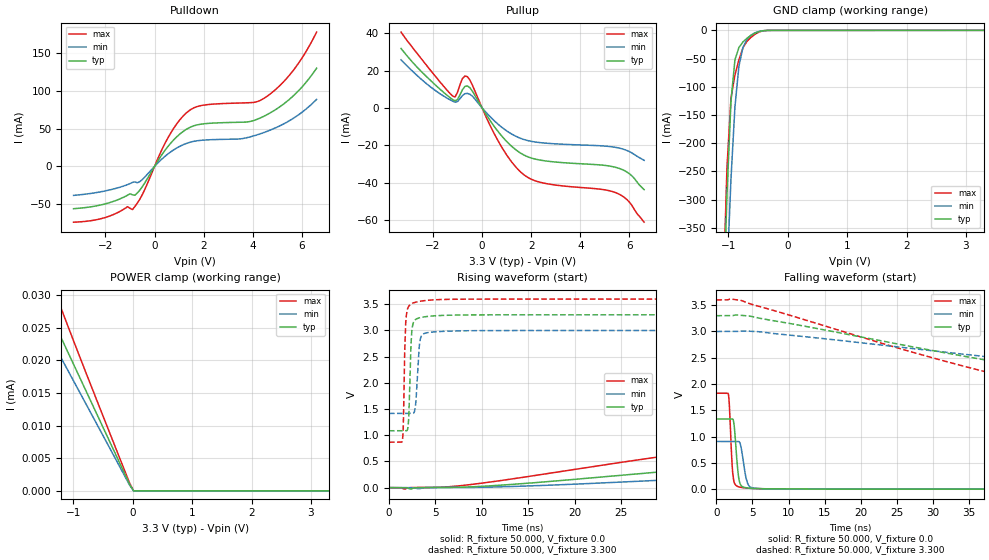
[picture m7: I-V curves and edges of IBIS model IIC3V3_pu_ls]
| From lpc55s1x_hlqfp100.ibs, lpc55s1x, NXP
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|   Model IIC3V3_pu_ls
[Model] IIC3V3_pu_ls
Model_type I/O
Polarity   Non-Inverting
Enable   Active-Low
Vinl =  0.990V
Vinh =  2.310V
Vmeas =  1.650V
Cref =  0.0F
Rref =  100.000
Vref =  0.0V
C_comp   2.367pF   2.322pF   2.392pF
C_comp_pullup   0.515pF   0.425pF   0.587pF
C_comp_pulldown   1.564pF   1.480pF   1.635pF
[Model Spec]
Vinh   2.310V   2.100V   2.520V
Vinl   0.990V   0.900V   1.080V
Vmeas   1.650V   1.500V   1.800V
Vref   0.0V   0.0V   0.0V
Cref   0.0F   0.0F   0.0F
Rref   100.000   100.000   100.000
[Temperature Range]   25.000   0.125k   -40.000
[Voltage Range]   3.300V   3.000V   3.600V
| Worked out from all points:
|   slope of the pulldown table from 0 to 0.495 V, typ, clamps not added: 20.4 ohm
|   slope of the pullup table from 0 to 0.495 V, typ, clamps not added: 49.8 ohm
|   GND clamp passes 1 mA (typ) near -0.43 V on its own axis
|   rising waveform, R_fixture 50.000, V_fixture 0.0: 20-80 % time 64.7ns typ, 78.1ns min, 51.2ns max; typ from 0.001 V to 1.33 V
|   rising waveform, R_fixture 50.000, V_fixture 3.300: 20-80 % time 237ps typ, 323ps min, 201ps max; typ from 1.09 V to 3.3 V
|   falling waveform, R_fixture 50.000, V_fixture 0.0: 20-80 % time 483ps typ, 657ps min, 379ps max; typ from 1.34 V to 0.001 V
|   falling waveform, R_fixture 50.000, V_fixture 3.300: 20-80 % time 50.7ns typ, 68.5ns min, 38.4ns max; typ from 3.3 V to 1.09 V
[Pulldown]
|Voltage   I(typ)   I(min)   I(max)
-3.3V     -56mA      -38.4mA    -73.87mA
-2.1V     -50.37mA   -33.07mA   -68.52mA
-1.1V     -38.15mA   -24.11mA   -53.37mA
-900mV    -37.61mA   -21.16mA   -57.18mA
-500mV    -26.92mA   -17.4mA    -37.43mA
500mV     24.51mA    15.34mA    35.14mA
1.2V      47.07mA    29.16mA    67.89mA
1.9V      55.94mA    34.55mA    80.54mA
3.8V      58.93mA    38.31mA    84.23mA
4.5V      67.15mA    45.39mA    91.04mA
5.6V      91.85mA    62.59mA    125mA
6.6V      130mA      88.72mA    177.8mA
[Pullup]
|Voltage   I(typ)   I(min)   I(max)
-3.3V     31.77mA    25.72mA    40.57mA
-2.2V     15.94mA    12.27mA    21.75mA
-1.2V     4.452mA    3.6mA      6.337mA
-1.1V     3.726mA    3.058mA    5.816mA
-800mV    9.696mA    6.594mA    15.7mA
-600mV    11.73mA    7.748mA    16.71mA
700mV     -13.46mA   -9.282mA   -18.76mA
1.7V      -25.21mA   -16.93mA   -35.78mA
2.6V      -28.44mA   -18.91mA   -40.52mA
5.5V      -32.06mA   -21.31mA   -45.71mA
6V        -35.26mA   -23.41mA   -50.46mA
6.6V      -43.77mA   -28.07mA   -61.22mA
[GND_clamp]
|Voltage   I(typ)   I(min)   I(max)
-3.3V     -10.05A    -9.18A     -11.33A
-1.089V   -516.6mA   -633.8mA   -475.1mA
-1.022V   -291.9mA   -436.4mA   -243.3mA
-955mV    -126.1mA   -264.1mA   -120.8mA
-888mV    -52.24mA   -135.7mA   -79.2mA
-821mV    -30.5mA    -63.74mA   -52.2mA
-754mV    -20.73mA   -30.74mA   -31.13mA
-687mV    -14.25mA   -16.02mA   -19.73mA
-553mV    -5.085mA   -4.563mA   -7.127mA
-419mV    -724uA     -765.2uA   -978.9uA
-285mV    -84.74uA   -88.26uA   -105.4uA
3.3V      0A         0A         0A
[POWER_clamp]
|Voltage   I(typ)   I(min)   I(max)
-3.3V     65.36uA    55.62uA    117.1uA
-1.792V   34.89uA    30.26uA    43.22uA
-1.725V   33.58uA    29.13uA    41.33uA
-1.524V   29.67uA    25.75uA    35.94uA
-1.323V   25.75uA    22.36uA    30.85uA
-1.256V   24.45uA    21.23uA    29.21uA
-921mV    17.94uA    15.59uA    21.23uA
-318mV    6.202uA    5.398uA    7.298uA
-50mV     976.9nA    858.9nA    1.15uA
17mV      0A         0A         0A
3.3V      0A         0A         0A
[Ramp]
| variable   typ   min   max
dV/dt_r   0.796/64.657n   0.535/78.119n   1.094/51.189n
dV/dt_f   1.328/50.692n   0.947/68.465n   1.639/38.378n
R_load = 50.000
[Rising Waveform]
R_fixture= 50.000
V_fixture= 0.0
V_fixture_min= 0.0
V_fixture_max= 0.0
|time   V(typ)   V(min)   V(max)
0s        843.5uV    916.9uV    820.9uV
1.74ns    921uV      917uV      -28.64mV
7.89ns    9.027mV    2.971mV    40.9mV
41.15ns   478.6mV    244.7mV    863.4mV
71.45ns   830.4mV    472.5mV    1.453V
84.34ns   982.7mV    552.4mV    1.619V
101.8ns   1.145V     655mV      1.728V
123.8ns   1.246V     770.7mV    1.785V
155.1ns   1.303V     851.6mV    1.813V
200ns     1.328V     891.7mV    1.824V
[Rising Waveform]
R_fixture= 50.000
V_fixture= 3.300
V_fixture_min= 3.000
V_fixture_max= 3.600
|time   V(typ)   V(min)   V(max)
0s        1.086V     1.417V     867.9mV
1.47ns    1.086V     1.417V     920.7mV
1.58ns    1.086V     1.417V     1.389V
1.75ns    1.086V     1.417V     2.906V
1.98ns    1.1V       1.417V     3.396V
2.56ns    3.101V     1.416V     3.522V
2.87ns    3.209V     1.569V     3.54V
3.37ns    3.246V     2.824V     3.559V
4.44ns    3.273V     2.966V     3.581V
200ns     3.3V       3V         3.6V
[Falling Waveform]
R_fixture= 50.000
V_fixture= 0.0
V_fixture_min= 0.0
V_fixture_max= 0.0
|time   V(typ)   V(min)   V(max)
0s        1.336V     908.4mV    1.826V
1.66ns    1.336V     908.4mV    1.808V
1.83ns    1.336V     908.4mV    1.518V
2.18ns    1.337V     908.4mV    457.9mV
2.47ns    1.201V     908.4mV    128.1mV
2.9ns     445.8mV    908.5mV    54.71mV
3.17ns    154.7mV    901.4mV    41.66mV
4.09ns    27.98mV    224.5mV    22.17mV
4.52ns    20.27mV    61.37mV    17.43mV
200ns     843.8uV    917.6uV    821uV
[Falling Waveform]
R_fixture= 50.000
V_fixture= 3.300
V_fixture_min= 3.000
V_fixture_max= 3.600
|time   V(typ)   V(min)   V(max)
0s        3.3V       3V         3.6V
3.36ns    3.307V     3.007V     3.593V
29.21ns   2.656V     2.643V     2.527V
49.05ns   2.196V     2.359V     1.841V
57.07ns   2.035V     2.258V     1.273V
66.1ns    1.793V     2.154V     1.026V
78.24ns   1.371V     2.024V     930.1mV
95.86ns   1.182V     1.724V     888.4mV
127.6ns   1.107V     1.491V     871.5mV
200ns     1.087V     1.422V     868mV
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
